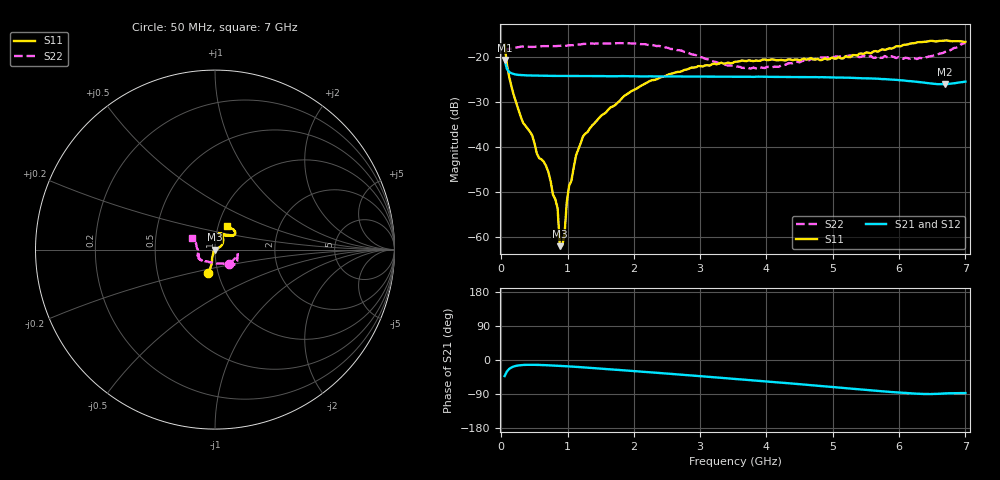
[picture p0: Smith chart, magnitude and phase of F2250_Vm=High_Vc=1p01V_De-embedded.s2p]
! Integrated Device Technology
! Corporate Headquarters
! 6024 Silver Creek Valley Road
! San Jose, CA 95138  USA
! Phone:  1-408-284-8200
! Toll Free:  1-800-223-1366
! Webpage:  http://www.idt.com/
! Timing and RF Division
! 515 Groton Road, Suite 102
! Westford, MA 01886-6024
! Device:  F2250
! Description: Voltage Variable RF Attenuator
! Frequency:  50.0 -  6000.00 MHz
! Package:  3x3 mm Thin QFN Plastic Package: 16 pin
! Ports:  2 RF, 3 DC
!  Pin  1  = GND
!  Pin  2  = NC
!  Pin  3  = RF1  = Port 1
!  Pin  4  = NC
!  Pin  5  = GND
!  Pin  6  = GND
!  Pin  7  = GND
!  Pin  8  = GND
!  Pin  9  = NC
!  Pin 10  = RF2  = Port 2
!  Pin 11  = NC
!  Pin 12  = GND
!  Pin 13  = GND
!  Pin 14  = VCNTRL
!  Pin 15  = VDD
!  Pin 16  = VMODE
! Vcntrl:  1.010 Volts
! Vmode:  +3.300 Volts
! Vdd:  +3.30  Volts
! Current:  1.327 mA
! Data:  The device was measured on a the F2250 evaluation board which has
!  individual transmission lines to the RF pins.  Data was collected
!  using a calibrated network analyzer.  The evaluation board was
!  de-embedded using a TRL calibration technique.
!  The reference plane is the edge of the package pin.
! Misc:  SN 10
!  Action Tracker AT0258
! Date Measured:  2014-11-26
! Date:  2015-10-15  MJV
! Note:
!  Integrated Device Technology supplies this data as a sample of measured
!  data at the package pin for this product.  Your particular data for this
!  product may vary.
!  Data was taken at 25 degrees C.
!  Integrated Device Technology reserves the right to change this data at anytime.
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# GHz S dB R 50
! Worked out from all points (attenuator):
!   201 points, 50 MHz to 7 GHz, reference 50 ohm
!   highest |S21| = -20.67 dB at 50 MHz (marker M1); lowest = -26.1 dB at 6.687 GHz (marker M2)
!   lowest |S11| = -62.1 dB at 884 MHz (marker M3), VSWR 1.00, Z = 49.9 - j0.00917 ohm
!   |S11| at or under -10 dB: start of sweep to end of sweep
!   |S22| runs from -22.6 to -16.9 dB; largest |S21 - S12| = 0.00023
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0.05  -17.28 -105.5  -20.67 -42.4  -20.68 -42.5  -18.99 -44.4
0.1195  -24.48 -106.1  -23.37 -23.5  -23.36 -23.5  -18.19 -16.3
0.29325  -33.28 -112.8  -24.03 -13.6  -24.03 -13.6  -17.73 -12.2
0.467  -37.47 -127.0  -24.16 -12.6  -24.17 -12.6  -17.79 -12.6
0.5365  -41.50 -128.7  -24.18 -12.9  -24.16 -12.9  -17.72 -14.1
0.71025  -45.58 -135.2  -24.21 -14.0  -24.20 -14.0  -17.59 -17.2
0.84925  -53.62 -169.1  -24.24 -15.2  -24.24 -15.2  -17.58 -20.2
0.884  -62.05 -173.3  -24.25 -15.5  -24.25 -15.5  -17.54 -21.2
0.91875  -61.88 99.6  -24.24 -15.9  -24.23 -15.9  -17.48 -21.9
0.9535  -59.48 -93.2  -24.23 -16.2  -24.24 -16.2  -17.58 -22.1
0.98825  -52.18 -27.8  -24.24 -16.6  -24.25 -16.6  -17.52 -22.7
1.023  -48.60 -4.4  -24.24 -16.9  -24.25 -16.9  -17.43 -22.9
1.05775  -47.50 4.1  -24.26 -17.3  -24.24 -17.3  -17.41 -23.1
1.12725  -41.88 10.6  -24.24 -18.1  -24.24 -18.1  -17.29 -24.6
1.2315  -37.70 15.0  -24.24 -19.3  -24.25 -19.3  -17.13 -26.6
1.857  -28.65 30.0  -24.28 -27.4  -24.29 -27.4  -16.95 -33.6
2.37825  -24.71 40.6  -24.34 -34.2  -24.35 -34.2  -17.56 -39.1
3.525  -21.06 68.9  -24.40 -49.9  -24.40 -49.9  -22.12 -81.0
4.7065  -20.56 70.6  -24.49 -67.0  -24.49 -67.0  -20.53 -140.6
5.85325  -18.09 39.1  -25.02 -84.1  -25.02 -84.2  -20.23 -160.9
6.68725  -16.37 46.9  -26.11 -88.3  -26.10 -88.4  -18.94 160.5
7  -16.67 61.9  -25.50 -87.2  -25.51 -87.3  -16.87 152.2
